(* Logix 5000 AddOnInstructionDefinition export Banner_Q5X_5000_Param_v4; software revision 33.00; part 2 of 3 *)
(* tags used below, declared in another part *)
   Q5X : Banner_Q5X_5000_v4;
   Port_Data : Banner_IOL_Port_v4;
   Port : DINT;
   Local_Control : DINT;
   Command_Being_Processed : BOOL;
   Update_Archive : BOOL;
   Index_Write_Inprocess : INT;
   Index_Write_Control : INT;
   Inprocess_Index : DINT;
(* Banner_Q5X_5000_Param_v4, continued *)

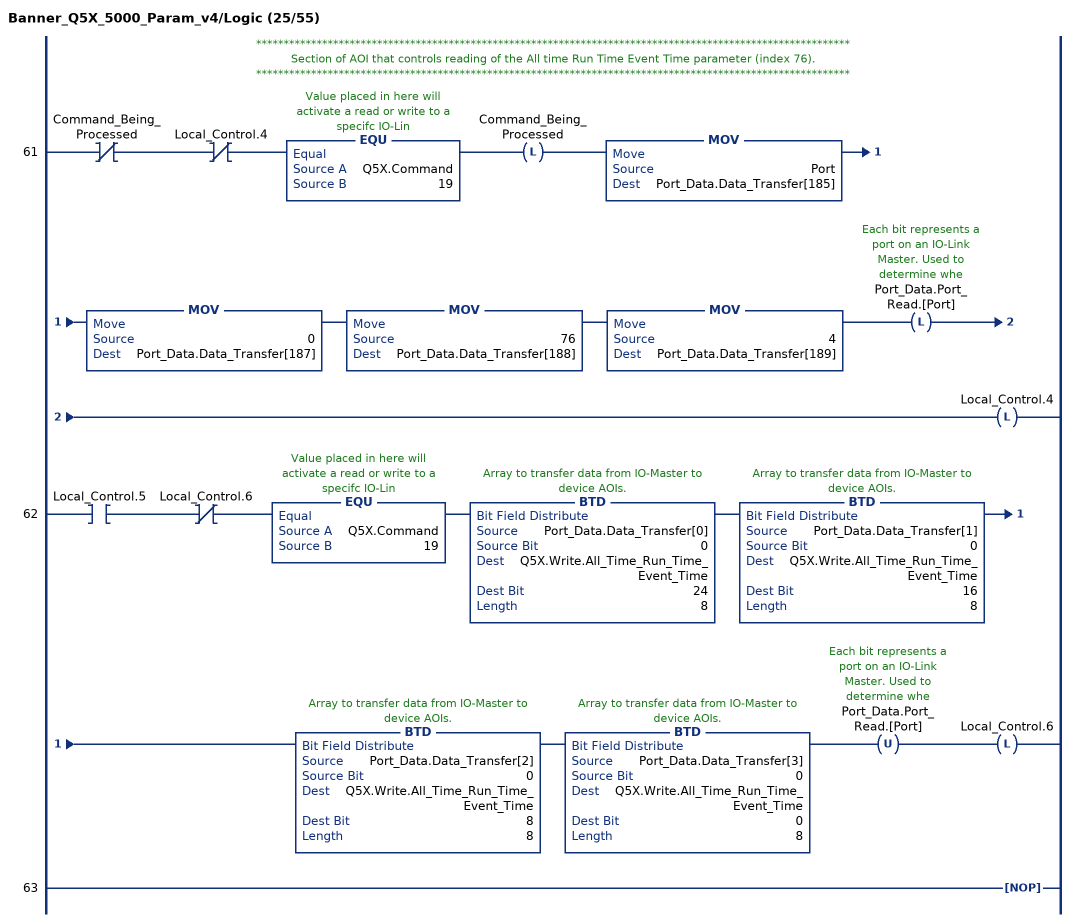
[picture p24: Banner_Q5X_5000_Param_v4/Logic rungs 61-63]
   // ************************************************************************************************************
   // Section of AOI that controls reading of the All time Run Time Event Time parameter (index 76).
   // ************************************************************************************************************
   61: XIO(Command_Being_Processed)XIO(Local_Control.4)EQU(Q5X.Command,19)OTL(Command_Being_Processed)MOV(Port,Port_Data.Data_Transfer[185])MOV(0,Port_Data.Data_Transfer[187])MOV(76,Port_Data.Data_Transfer[188])MOV(4,Port_Data.Data_Transfer[189])OTL(Port_Data.Port_Read.[Port])OTL(Local_Control.4);
   62: XIC(Local_Control.5)XIO(Local_Control.6)EQU(Q5X.Command,19)BTD(Port_Data.Data_Transfer[0],0,Q5X.Write.All_Time_Run_Time_Event_Time,24,8)BTD(Port_Data.Data_Transfer[1],0,Q5X.Write.All_Time_Run_Time_Event_Time,16,8)BTD(Port_Data.Data_Transfer[2],0,Q5X.Write.All_Time_Run_Time_Event_Time,8,8)BTD(Port_Data.Data_Transfer[3],0,Q5X.Write.All_Time_Run_Time_Event_Time,0,8)OTU(Port_Data.Port_Read.[Port])OTL(Local_Control.6);
   63: NOP();
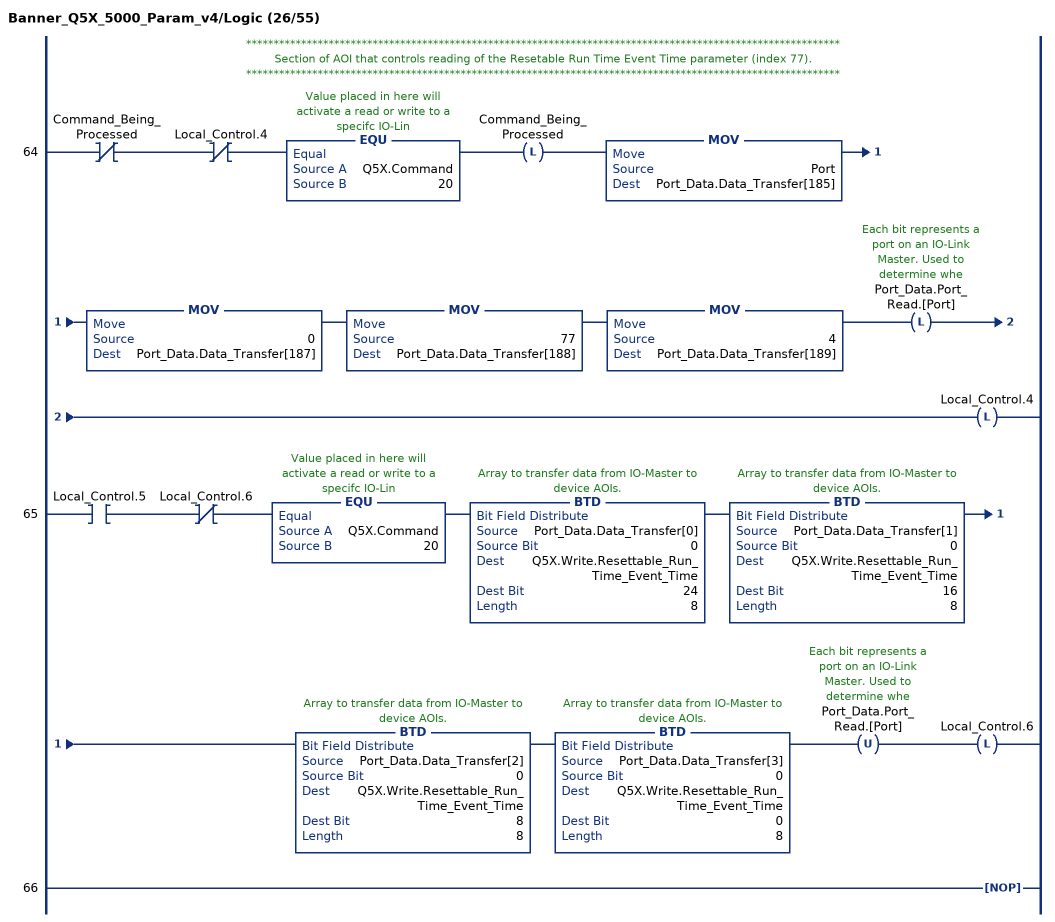
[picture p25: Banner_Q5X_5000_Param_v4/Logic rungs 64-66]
   // ************************************************************************************************************
   // Section of AOI that controls reading of the Resetable Run Time Event Time parameter (index 77).
   // ************************************************************************************************************
   64: XIO(Command_Being_Processed)XIO(Local_Control.4)EQU(Q5X.Command,20)OTL(Command_Being_Processed)MOV(Port,Port_Data.Data_Transfer[185])MOV(0,Port_Data.Data_Transfer[187])MOV(77,Port_Data.Data_Transfer[188])MOV(4,Port_Data.Data_Transfer[189])OTL(Port_Data.Port_Read.[Port])OTL(Local_Control.4);
   65: XIC(Local_Control.5)XIO(Local_Control.6)EQU(Q5X.Command,20)BTD(Port_Data.Data_Transfer[0],0,Q5X.Write.Resettable_Run_Time_Event_Time,24,8)BTD(Port_Data.Data_Transfer[1],0,Q5X.Write.Resettable_Run_Time_Event_Time,16,8)BTD(Port_Data.Data_Transfer[2],0,Q5X.Write.Resettable_Run_Time_Event_Time,8,8)BTD(Port_Data.Data_Transfer[3],0,Q5X.Write.Resettable_Run_Time_Event_Time,0,8)OTU(Port_Data.Port_Read.[Port])OTL(Local_Control.6);
   66: NOP();
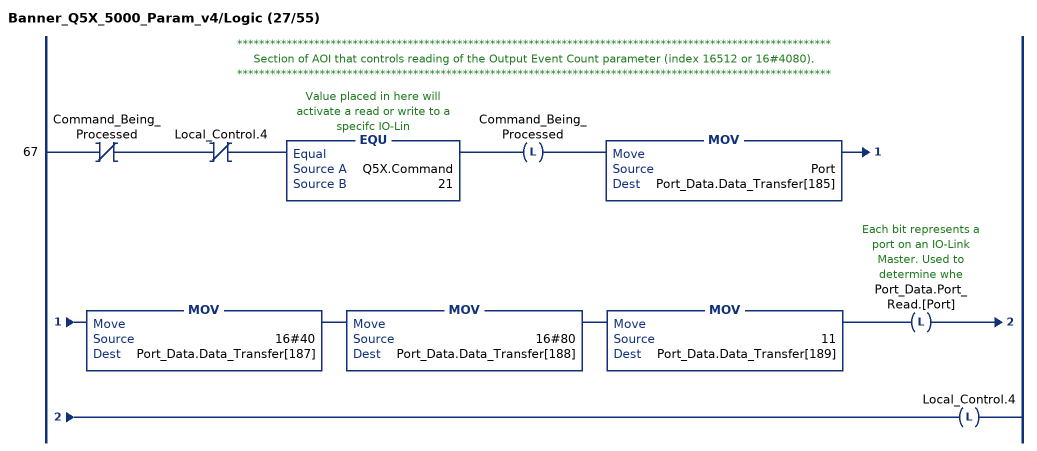
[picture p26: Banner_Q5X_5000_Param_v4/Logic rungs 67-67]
   // ************************************************************************************************************
   // Section of AOI that controls reading of the Output Event Count parameter (index 16512 or 16#4080).
   // ************************************************************************************************************
   67: XIO(Command_Being_Processed)XIO(Local_Control.4)EQU(Q5X.Command,21)OTL(Command_Being_Processed)MOV(Port,Port_Data.Data_Transfer[185])MOV(16#40,Port_Data.Data_Transfer[187])MOV(16#80,Port_Data.Data_Transfer[188])MOV(11,Port_Data.Data_Transfer[189])OTL(Port_Data.Port_Read.[Port])OTL(Local_Control.4);
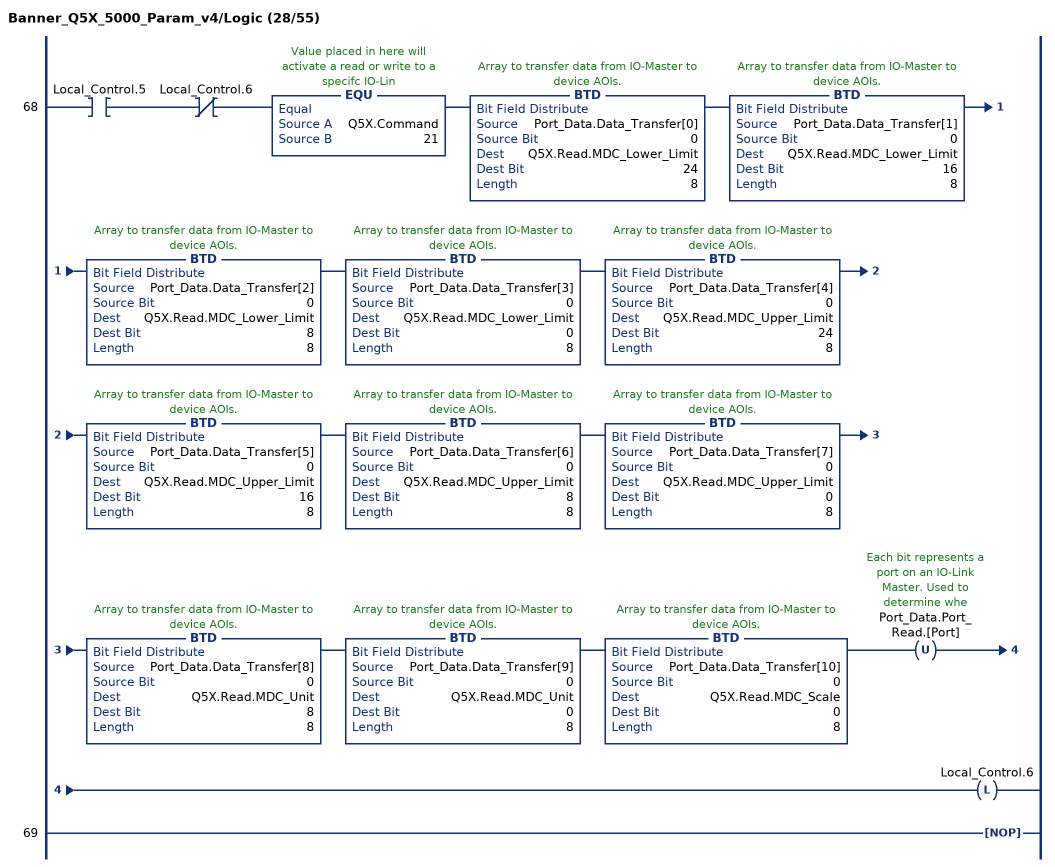
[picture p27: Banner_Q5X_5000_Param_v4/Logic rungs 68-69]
   68: XIC(Local_Control.5)XIO(Local_Control.6)EQU(Q5X.Command,21)BTD(Port_Data.Data_Transfer[0],0,Q5X.Read.MDC_Lower_Limit,24,8)BTD(Port_Data.Data_Transfer[1],0,Q5X.Read.MDC_Lower_Limit,16,8)BTD(Port_Data.Data_Transfer[2],0,Q5X.Read.MDC_Lower_Limit,8,8)BTD(Port_Data.Data_Transfer[3],0,Q5X.Read.MDC_Lower_Limit,0,8)BTD(Port_Data.Data_Transfer[4],0,Q5X.Read.MDC_Upper_Limit,24,8)BTD(Port_Data.Data_Transfer[5],0,Q5X.Read.MDC_Upper_Limit,16,8)BTD(Port_Data.Data_Transfer[6],0,Q5X.Read.MDC_Upper_Limit,8,8)BTD(Port_Data.Data_Transfer[7],0,Q5X.Read.MDC_Upper_Limit,0,8)BTD(Port_Data.Data_Transfer[8],0,Q5X.Read.MDC_Unit,8,8)BTD(Port_Data.Data_Transfer[9],0,Q5X.Read.MDC_Unit,0,8)BTD(Port_Data.Data_Transfer[10],0,Q5X.Read.MDC_Scale,0,8)OTU(Port_Data.Port_Read.[Port])OTL(Local_Control.6);
   69: NOP();
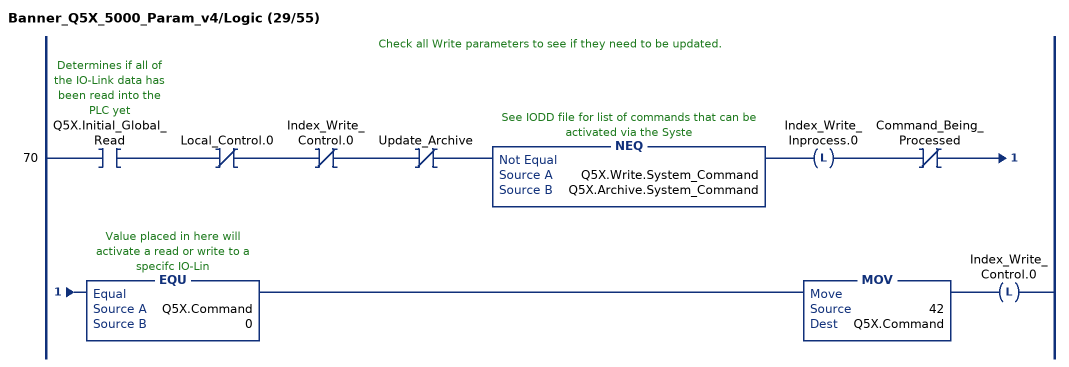
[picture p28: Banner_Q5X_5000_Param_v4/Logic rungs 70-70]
   // Check all Write parameters to see if they need to be updated.
   70: XIC(Q5X.Initial_Global_Read)XIO(Local_Control.0)XIO(Index_Write_Control.0)XIO(Update_Archive)NEQ(Q5X.Write.System_Command,Q5X.Archive.System_Command)OTL(Index_Write_Inprocess.0)XIO(Command_Being_Processed)EQU(Q5X.Command,0)MOV(42,Q5X.Command)OTL(Index_Write_Control.0);
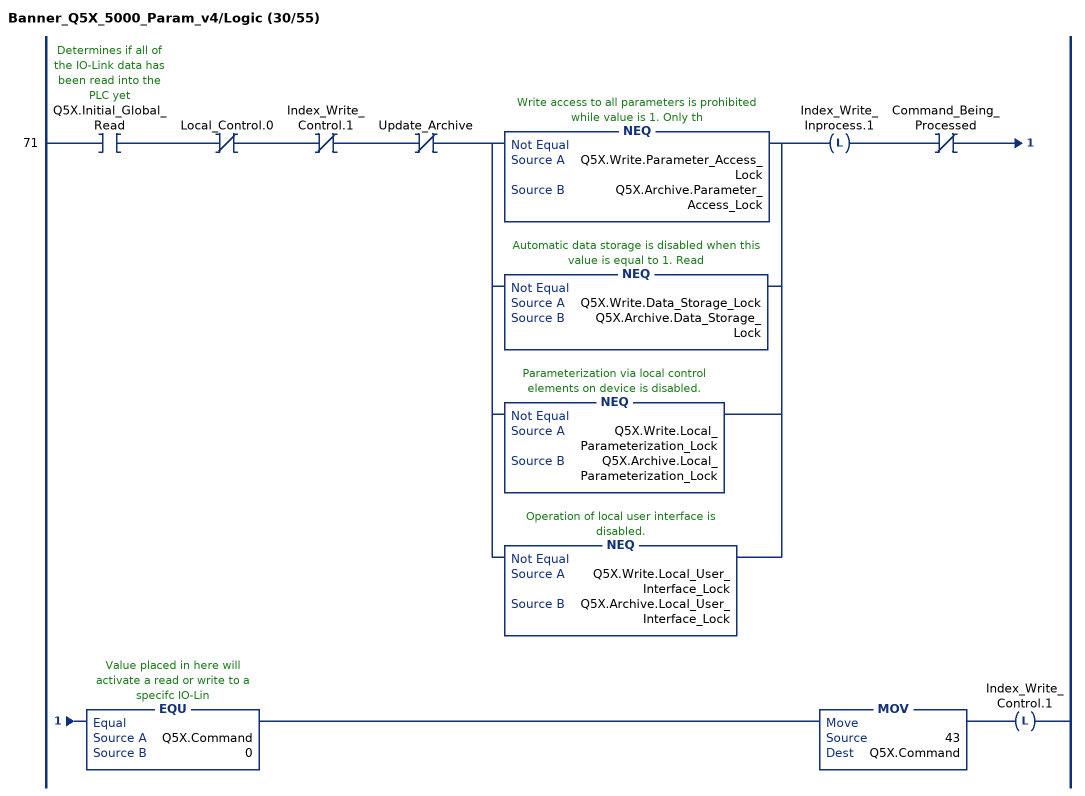
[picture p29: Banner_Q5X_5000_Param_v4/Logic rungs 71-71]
   71: XIC(Q5X.Initial_Global_Read)XIO(Local_Control.0)XIO(Index_Write_Control.1)XIO(Update_Archive)[NEQ(Q5X.Write.Parameter_Access_Lock,Q5X.Archive.Parameter_Access_Lock) ,NEQ(Q5X.Write.Data_Storage_Lock,Q5X.Archive.Data_Storage_Lock) ,NEQ(Q5X.Write.Local_Parameterization_Lock,Q5X.Archive.Local_Parameterization_Lock) ,NEQ(Q5X.Write.Local_User_Interface_Lock,Q5X.Archive.Local_User_Interface_Lock) ]OTL(Index_Write_Inprocess.1)XIO(Command_Being_Processed)EQU(Q5X.Command,0)MOV(43,Q5X.Command)OTL(Index_Write_Control.1);
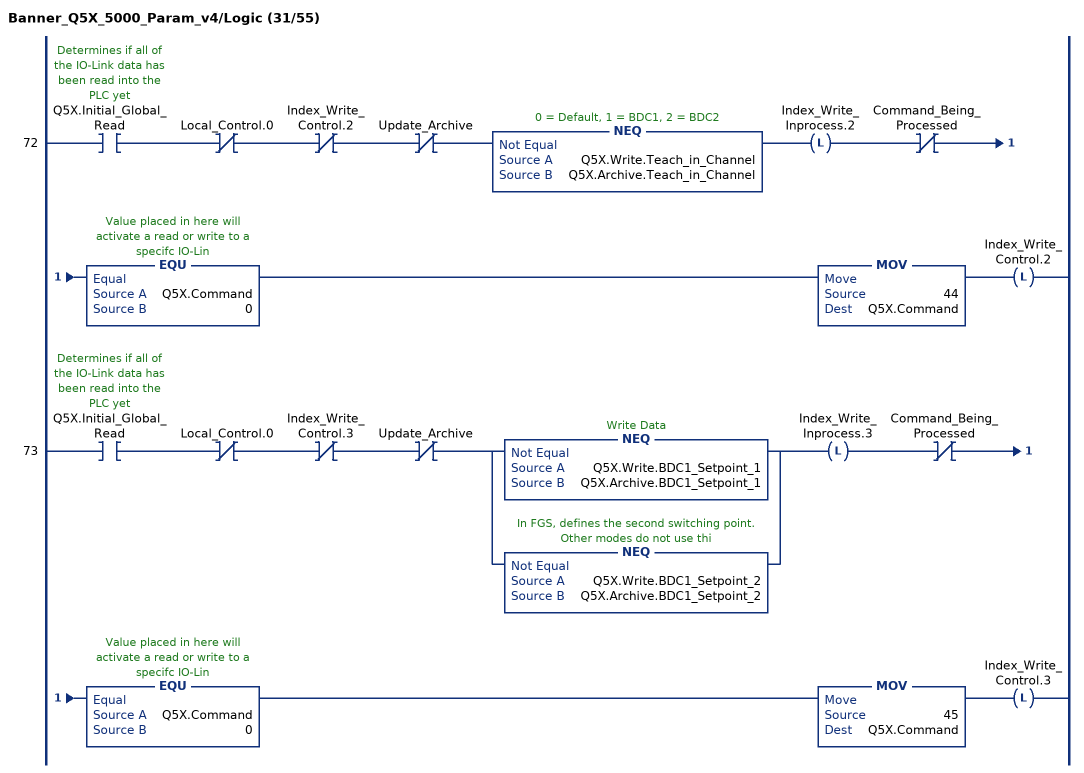
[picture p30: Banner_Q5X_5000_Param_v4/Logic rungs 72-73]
   72: XIC(Q5X.Initial_Global_Read)XIO(Local_Control.0)XIO(Index_Write_Control.2)XIO(Update_Archive)NEQ(Q5X.Write.Teach_in_Channel,Q5X.Archive.Teach_in_Channel)OTL(Index_Write_Inprocess.2)XIO(Command_Being_Processed)EQU(Q5X.Command,0)MOV(44,Q5X.Command)OTL(Index_Write_Control.2);
   73: XIC(Q5X.Initial_Global_Read)XIO(Local_Control.0)XIO(Index_Write_Control.3)XIO(Update_Archive)[NEQ(Q5X.Write.BDC1_Setpoint_1,Q5X.Archive.BDC1_Setpoint_1) ,NEQ(Q5X.Write.BDC1_Setpoint_2,Q5X.Archive.BDC1_Setpoint_2) ]OTL(Index_Write_Inprocess.3)XIO(Command_Being_Processed)EQU(Q5X.Command,0)MOV(45,Q5X.Command)OTL(Index_Write_Control.3);
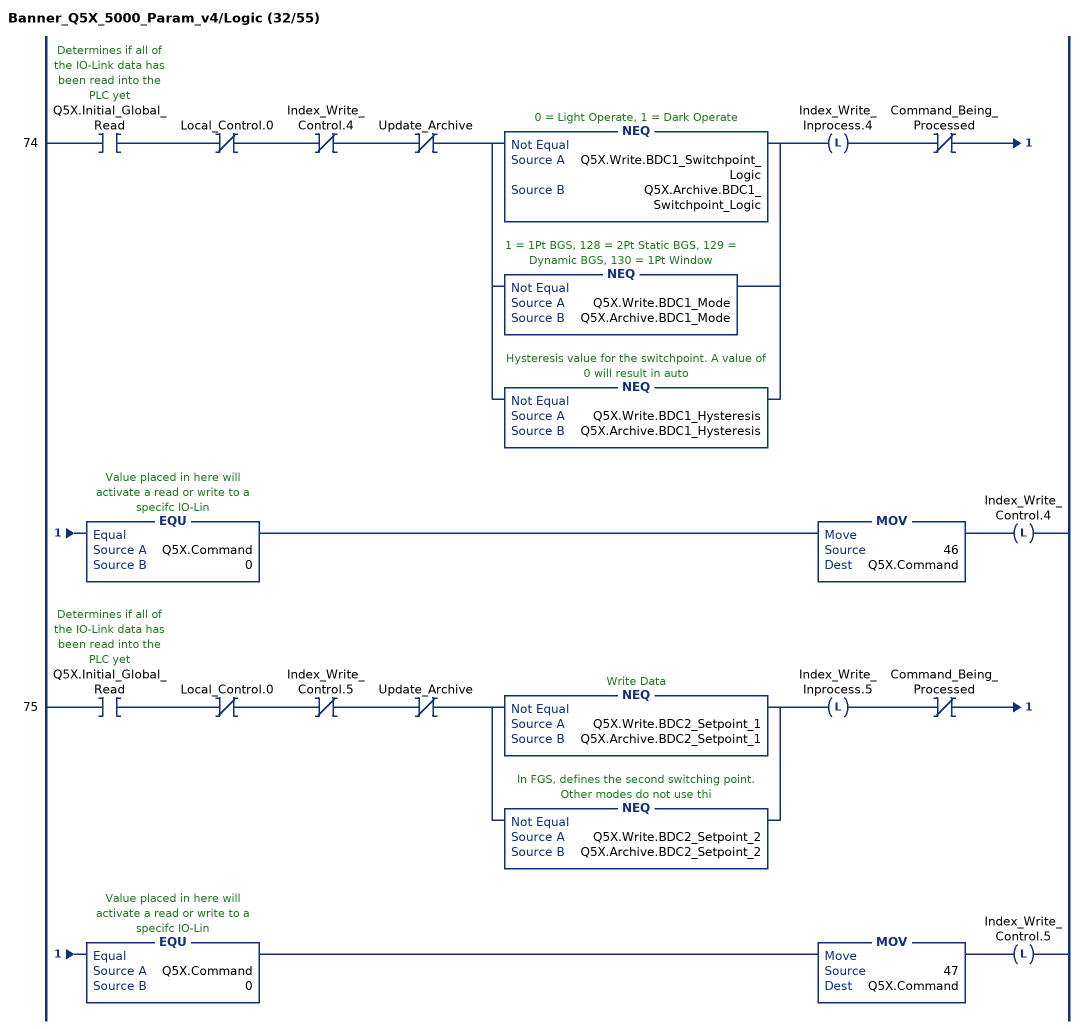
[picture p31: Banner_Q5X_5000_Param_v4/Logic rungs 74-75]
   74: XIC(Q5X.Initial_Global_Read)XIO(Local_Control.0)XIO(Index_Write_Control.4)XIO(Update_Archive)[NEQ(Q5X.Write.BDC1_Switchpoint_Logic,Q5X.Archive.BDC1_Switchpoint_Logic) ,NEQ(Q5X.Write.BDC1_Mode,Q5X.Archive.BDC1_Mode) ,NEQ(Q5X.Write.BDC1_Hysteresis,Q5X.Archive.BDC1_Hysteresis) ]OTL(Index_Write_Inprocess.4)XIO(Command_Being_Processed)EQU(Q5X.Command,0)MOV(46,Q5X.Command)OTL(Index_Write_Control.4);
   75: XIC(Q5X.Initial_Global_Read)XIO(Local_Control.0)XIO(Index_Write_Control.5)XIO(Update_Archive)[NEQ(Q5X.Write.BDC2_Setpoint_1,Q5X.Archive.BDC2_Setpoint_1) ,NEQ(Q5X.Write.BDC2_Setpoint_2,Q5X.Archive.BDC2_Setpoint_2) ]OTL(Index_Write_Inprocess.5)XIO(Command_Being_Processed)EQU(Q5X.Command,0)MOV(47,Q5X.Command)OTL(Index_Write_Control.5);
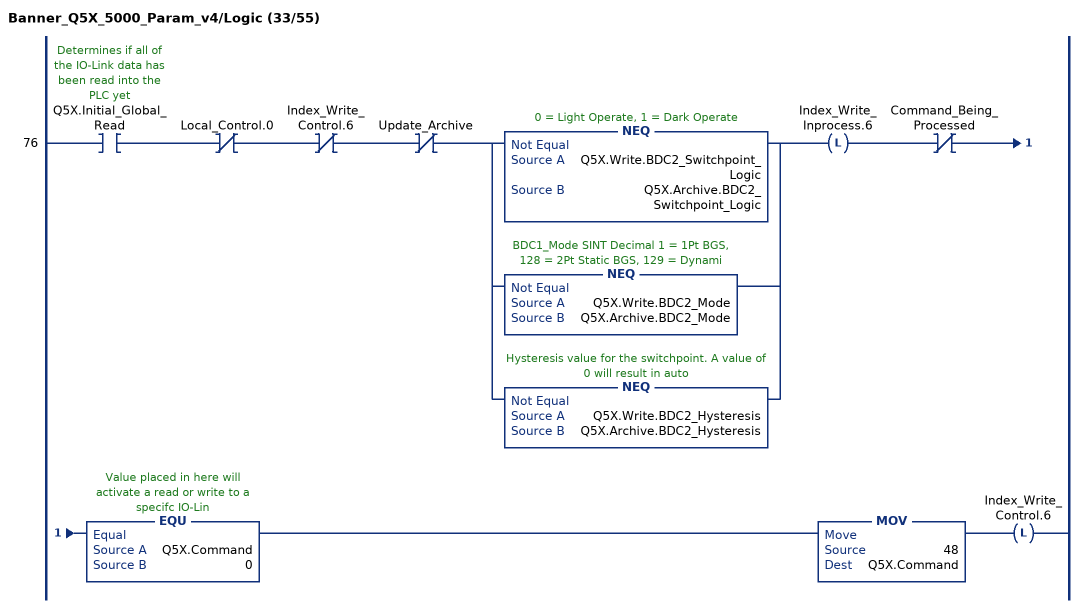
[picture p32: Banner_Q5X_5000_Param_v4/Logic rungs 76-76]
   76: XIC(Q5X.Initial_Global_Read)XIO(Local_Control.0)XIO(Index_Write_Control.6)XIO(Update_Archive)[NEQ(Q5X.Write.BDC2_Switchpoint_Logic,Q5X.Archive.BDC2_Switchpoint_Logic) ,NEQ(Q5X.Write.BDC2_Mode,Q5X.Archive.BDC2_Mode) ,NEQ(Q5X.Write.BDC2_Hysteresis,Q5X.Archive.BDC2_Hysteresis) ]OTL(Index_Write_Inprocess.6)XIO(Command_Being_Processed)EQU(Q5X.Command,0)MOV(48,Q5X.Command)OTL(Index_Write_Control.6);
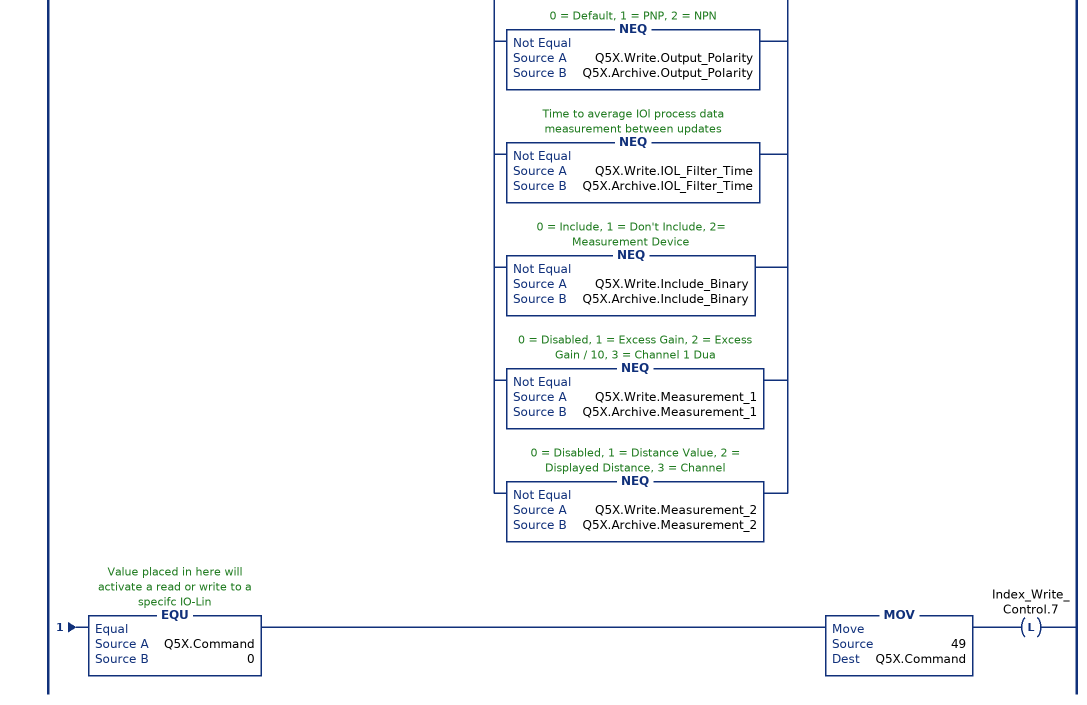
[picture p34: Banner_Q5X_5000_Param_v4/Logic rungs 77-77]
   77: XIC(Q5X.Initial_Global_Read)XIO(Local_Control.0)XIO(Index_Write_Control.7)XIO(Update_Archive)[NEQ(Q5X.Write.Response_Speed,Q5X.Archive.Response_Speed) ,NEQ(Q5X.Write.Gain,Q5X.Archive.Gain) ,NEQ(Q5X.Write.Secondary_Output_Mode,Q5X.Archive.Secondary_Output_Mode) ,NEQ(Q5X.Write.Zero_Reference_Location,Q5X.Archive.Zero_Reference_Location) ,NEQ(Q5X.Write.Shift_Zero_after_Teach,Q5X.Archive.Shift_Zero_after_Teach) ,NEQ(Q5X.Write.Display_Read,Q5X.Archive.Display_Read) ,NEQ(Q5X.Write.Display_Units,Q5X.Archive.Display_Units) ,NEQ(Q5X.Write.Pushbutton_Lockout,Q5X.Archive.Pushbutton_Lockout) ,NEQ(Q5X.Write.Output_Polarity,Q5X.Archive.Output_Polarity) ,NEQ(Q5X.Write.IOL_Filter_Time,Q5X.Archive.IOL_Filter_Time) ,NEQ(Q5X.Write.Include_Binary,Q5X.Archive.Include_Binary) ,NEQ(Q5X.Write.Measurement_1,Q5X.Archive.Measurement_1) ,NEQ(Q5X.Write.Measurement_2,Q5X.Archive.Measurement_2) ]OTL(Index_Write_Inprocess.7)XIO(Command_Being_Processed)EQU(Q5X.Command,0)MOV(49,Q5X.Command)OTL(Index_Write_Control.7);
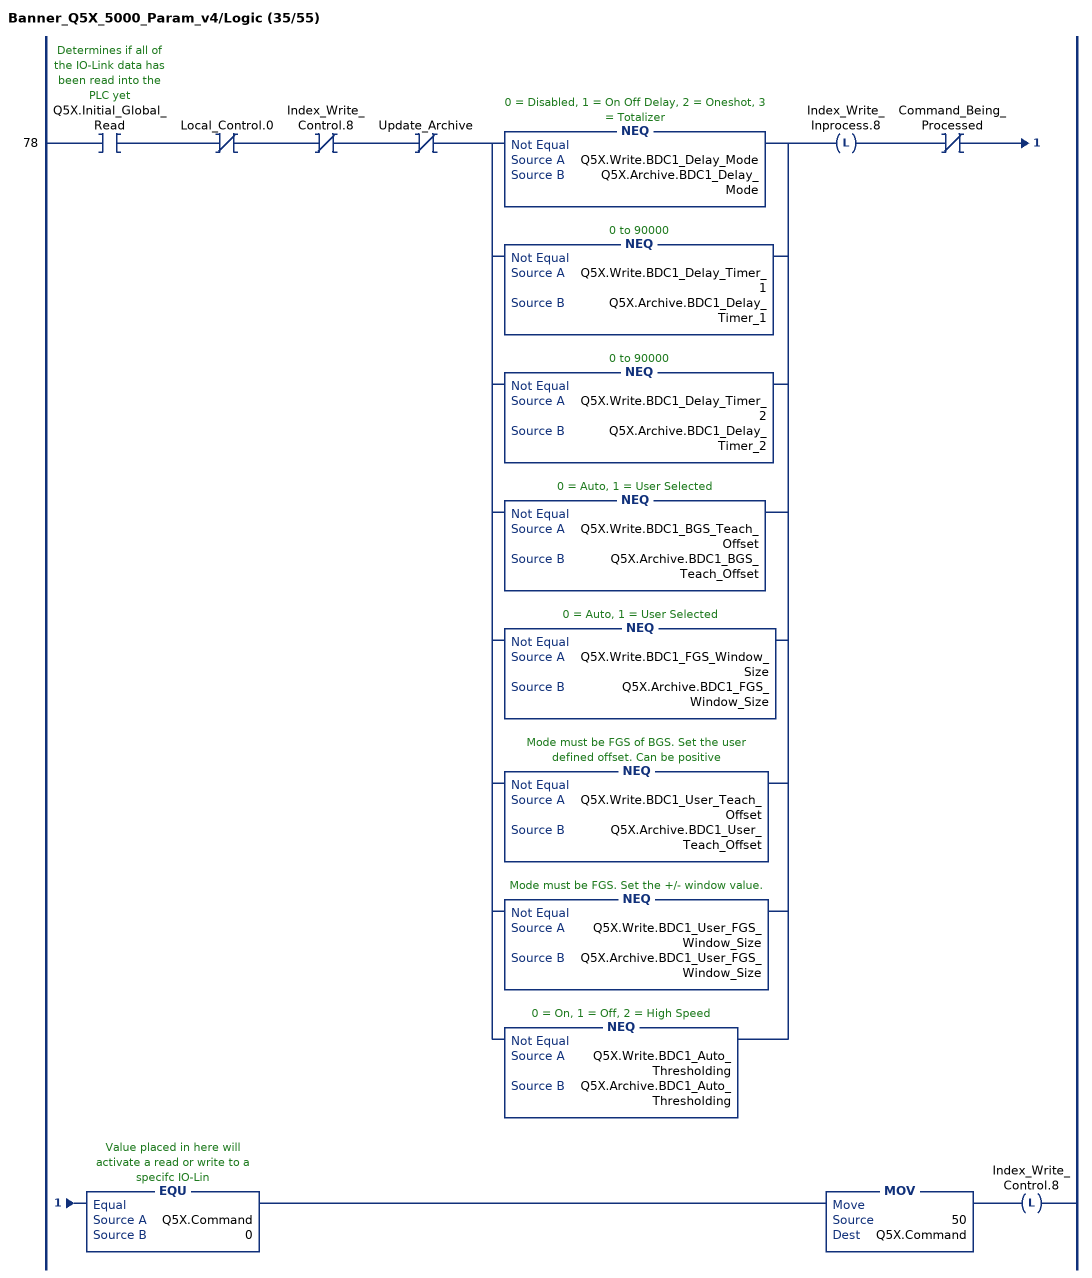
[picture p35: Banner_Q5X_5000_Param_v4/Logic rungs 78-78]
   78: XIC(Q5X.Initial_Global_Read)XIO(Local_Control.0)XIO(Index_Write_Control.8)XIO(Update_Archive)[NEQ(Q5X.Write.BDC1_Delay_Mode,Q5X.Archive.BDC1_Delay_Mode) ,NEQ(Q5X.Write.BDC1_Delay_Timer_1,Q5X.Archive.BDC1_Delay_Timer_1) ,NEQ(Q5X.Write.BDC1_Delay_Timer_2,Q5X.Archive.BDC1_Delay_Timer_2) ,NEQ(Q5X.Write.BDC1_BGS_Teach_Offset,Q5X.Archive.BDC1_BGS_Teach_Offset) ,NEQ(Q5X.Write.BDC1_FGS_Window_Size,Q5X.Archive.BDC1_FGS_Window_Size) ,NEQ(Q5X.Write.BDC1_User_Teach_Offset,Q5X.Archive.BDC1_User_Teach_Offset) ,NEQ(Q5X.Write.BDC1_User_FGS_Window_Size,Q5X.Archive.BDC1_User_FGS_Window_Size) ,NEQ(Q5X.Write.BDC1_Auto_Thresholding,Q5X.Archive.BDC1_Auto_Thresholding) ]OTL(Index_Write_Inprocess.8)XIO(Command_Being_Processed)EQU(Q5X.Command,0)MOV(50,Q5X.Command)OTL(Index_Write_Control.8);
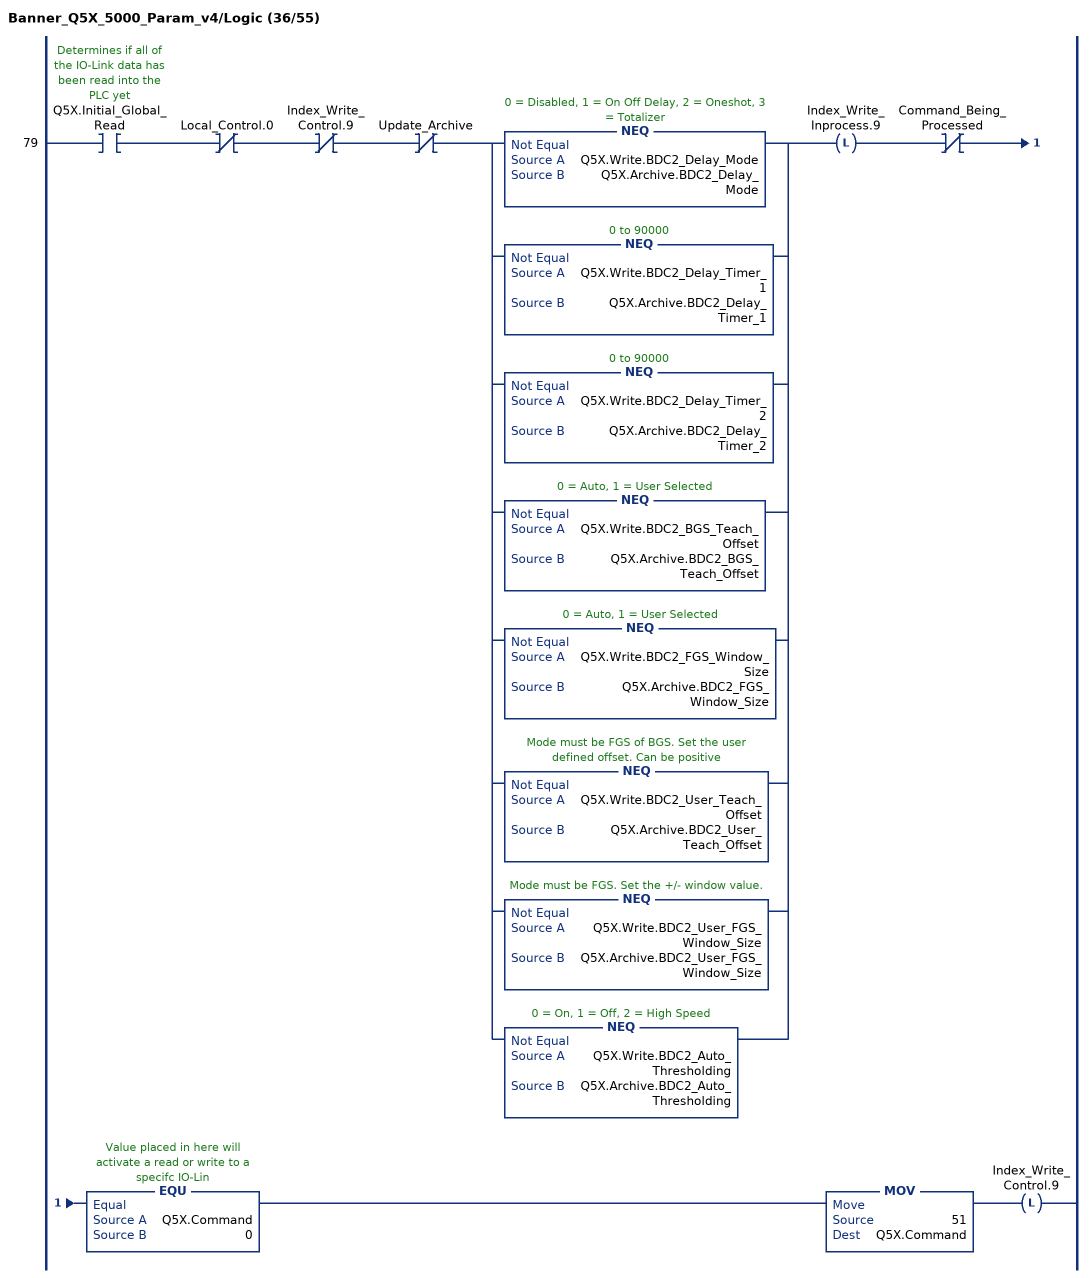
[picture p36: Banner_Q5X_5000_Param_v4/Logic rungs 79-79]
   79: XIC(Q5X.Initial_Global_Read)XIO(Local_Control.0)XIO(Index_Write_Control.9)XIO(Update_Archive)[NEQ(Q5X.Write.BDC2_Delay_Mode,Q5X.Archive.BDC2_Delay_Mode) ,NEQ(Q5X.Write.BDC2_Delay_Timer_1,Q5X.Archive.BDC2_Delay_Timer_1) ,NEQ(Q5X.Write.BDC2_Delay_Timer_2,Q5X.Archive.BDC2_Delay_Timer_2) ,NEQ(Q5X.Write.BDC2_BGS_Teach_Offset,Q5X.Archive.BDC2_BGS_Teach_Offset) ,NEQ(Q5X.Write.BDC2_FGS_Window_Size,Q5X.Archive.BDC2_FGS_Window_Size) ,NEQ(Q5X.Write.BDC2_User_Teach_Offset,Q5X.Archive.BDC2_User_Teach_Offset) ,NEQ(Q5X.Write.BDC2_User_FGS_Window_Size,Q5X.Archive.BDC2_User_FGS_Window_Size) ,NEQ(Q5X.Write.BDC2_Auto_Thresholding,Q5X.Archive.BDC2_Auto_Thresholding) ]OTL(Index_Write_Inprocess.9)XIO(Command_Being_Processed)EQU(Q5X.Command,0)MOV(51,Q5X.Command)OTL(Index_Write_Control.9);
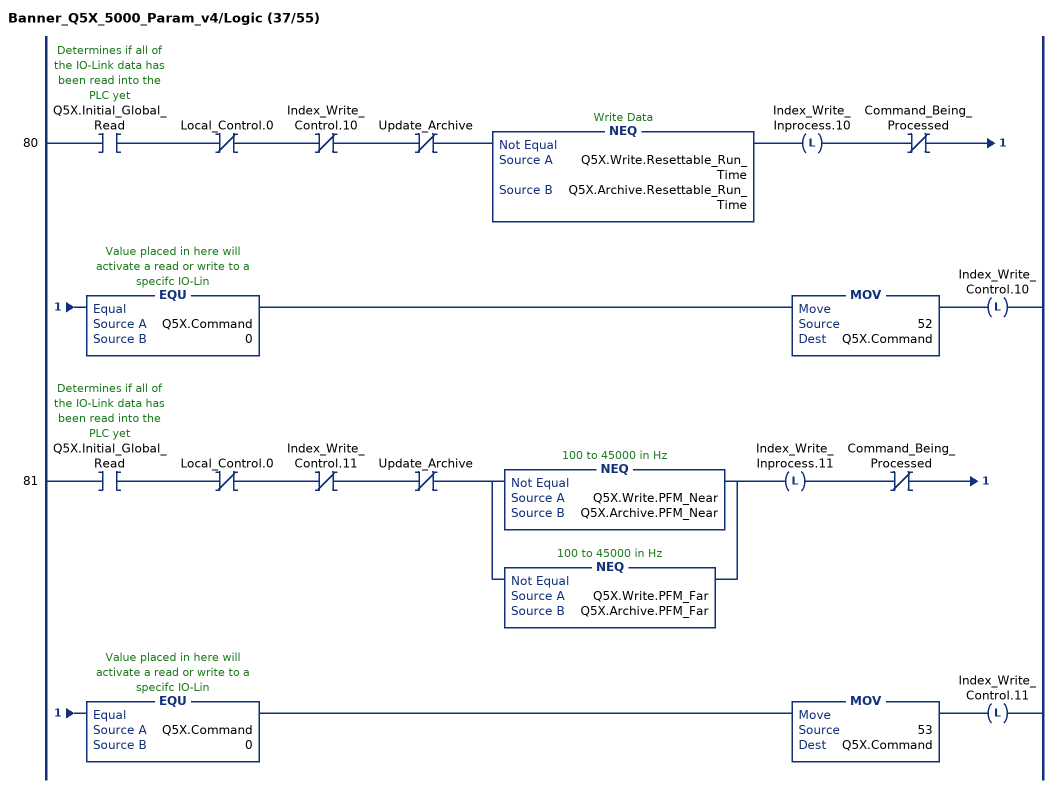
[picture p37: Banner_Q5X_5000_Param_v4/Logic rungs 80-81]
   80: XIC(Q5X.Initial_Global_Read)XIO(Local_Control.0)XIO(Index_Write_Control.10)XIO(Update_Archive)NEQ(Q5X.Write.Resettable_Run_Time,Q5X.Archive.Resettable_Run_Time)OTL(Index_Write_Inprocess.10)XIO(Command_Being_Processed)EQU(Q5X.Command,0)MOV(52,Q5X.Command)OTL(Index_Write_Control.10);
   81: XIC(Q5X.Initial_Global_Read)XIO(Local_Control.0)XIO(Index_Write_Control.11)XIO(Update_Archive)[NEQ(Q5X.Write.PFM_Near,Q5X.Archive.PFM_Near) ,NEQ(Q5X.Write.PFM_Far,Q5X.Archive.PFM_Far) ]OTL(Index_Write_Inprocess.11)XIO(Command_Being_Processed)EQU(Q5X.Command,0)MOV(53,Q5X.Command)OTL(Index_Write_Control.11);
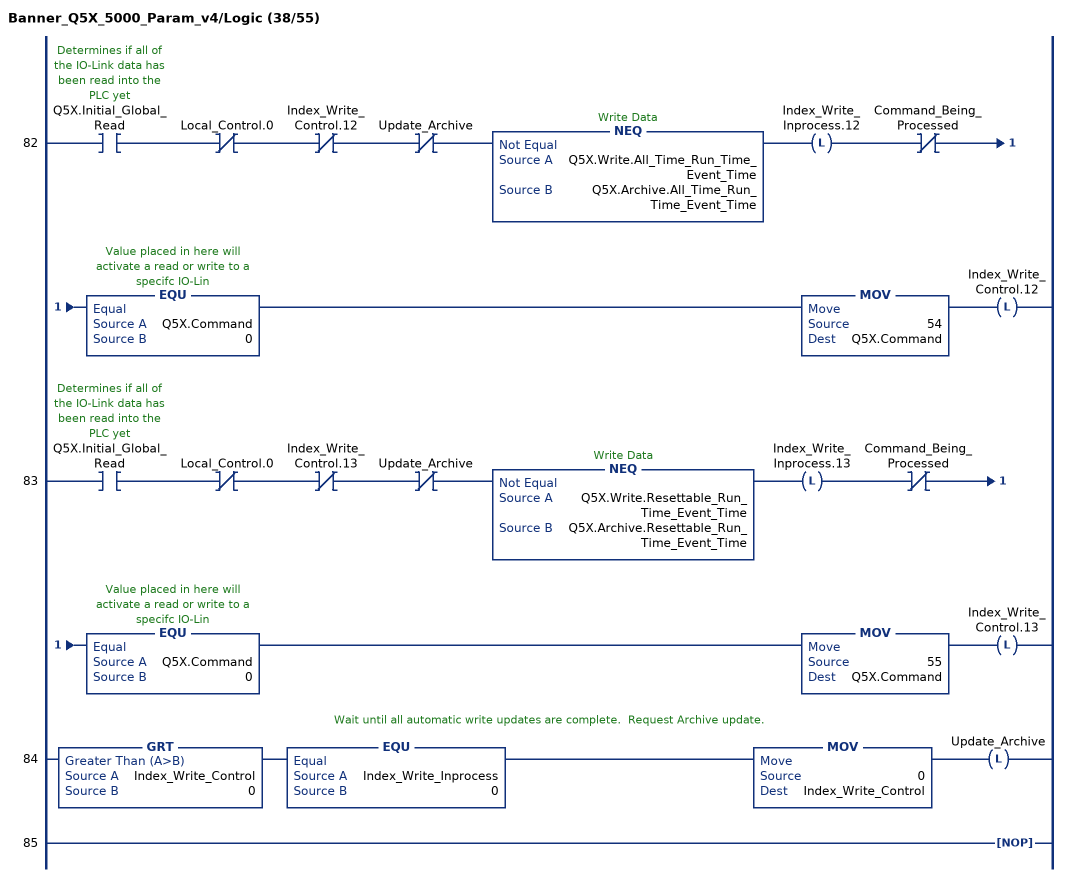
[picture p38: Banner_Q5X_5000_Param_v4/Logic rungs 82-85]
   82: XIC(Q5X.Initial_Global_Read)XIO(Local_Control.0)XIO(Index_Write_Control.12)XIO(Update_Archive)NEQ(Q5X.Write.All_Time_Run_Time_Event_Time,Q5X.Archive.All_Time_Run_Time_Event_Time)OTL(Index_Write_Inprocess.12)XIO(Command_Being_Processed)EQU(Q5X.Command,0)MOV(54,Q5X.Command)OTL(Index_Write_Control.12);
   83: XIC(Q5X.Initial_Global_Read)XIO(Local_Control.0)XIO(Index_Write_Control.13)XIO(Update_Archive)NEQ(Q5X.Write.Resettable_Run_Time_Event_Time,Q5X.Archive.Resettable_Run_Time_Event_Time)OTL(Index_Write_Inprocess.13)XIO(Command_Being_Processed)EQU(Q5X.Command,0)MOV(55,Q5X.Command)OTL(Index_Write_Control.13);
   // Wait until all automatic write updates are complete.  Request Archive update.
   84: GRT(Index_Write_Control,0)EQU(Index_Write_Inprocess,0)MOV(0,Index_Write_Control)OTL(Update_Archive);
   85: NOP();
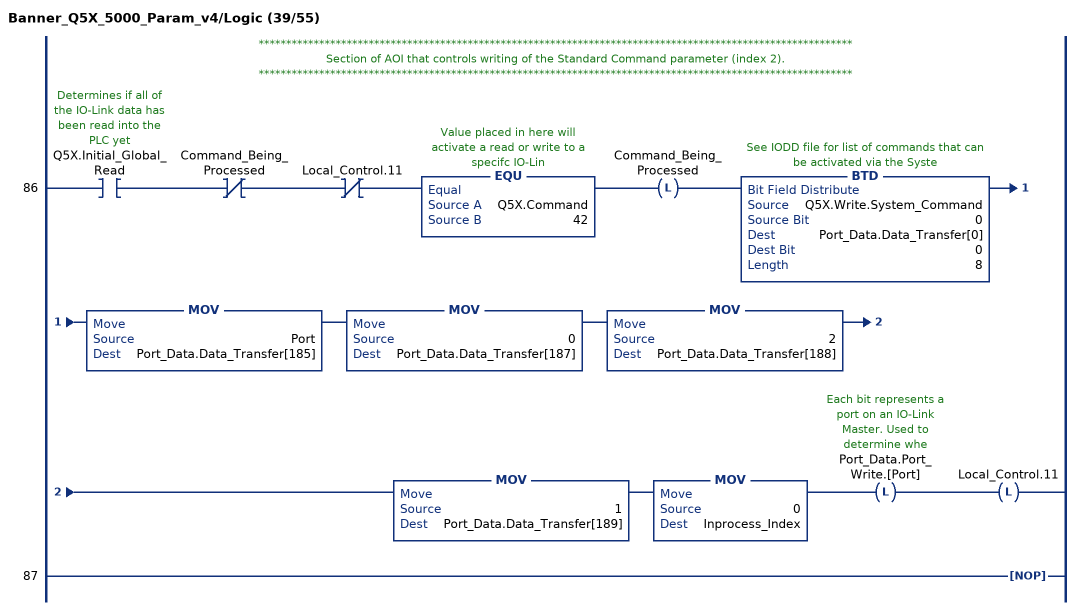
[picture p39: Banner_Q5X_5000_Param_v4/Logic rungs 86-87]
   // ************************************************************************************************************
   // Section of AOI that controls writing of the Standard Command parameter (index 2).
   // ************************************************************************************************************
   86: XIC(Q5X.Initial_Global_Read)XIO(Command_Being_Processed)XIO(Local_Control.11)EQU(Q5X.Command,42)OTL(Command_Being_Processed)BTD(Q5X.Write.System_Command,0,Port_Data.Data_Transfer[0],0,8)MOV(Port,Port_Data.Data_Transfer[185])MOV(0,Port_Data.Data_Transfer[187])MOV(2,Port_Data.Data_Transfer[188])MOV(1,Port_Data.Data_Transfer[189])MOV(0,Inprocess_Index)OTL(Port_Data.Port_Write.[Port])OTL(Local_Control.11);
   87: NOP();
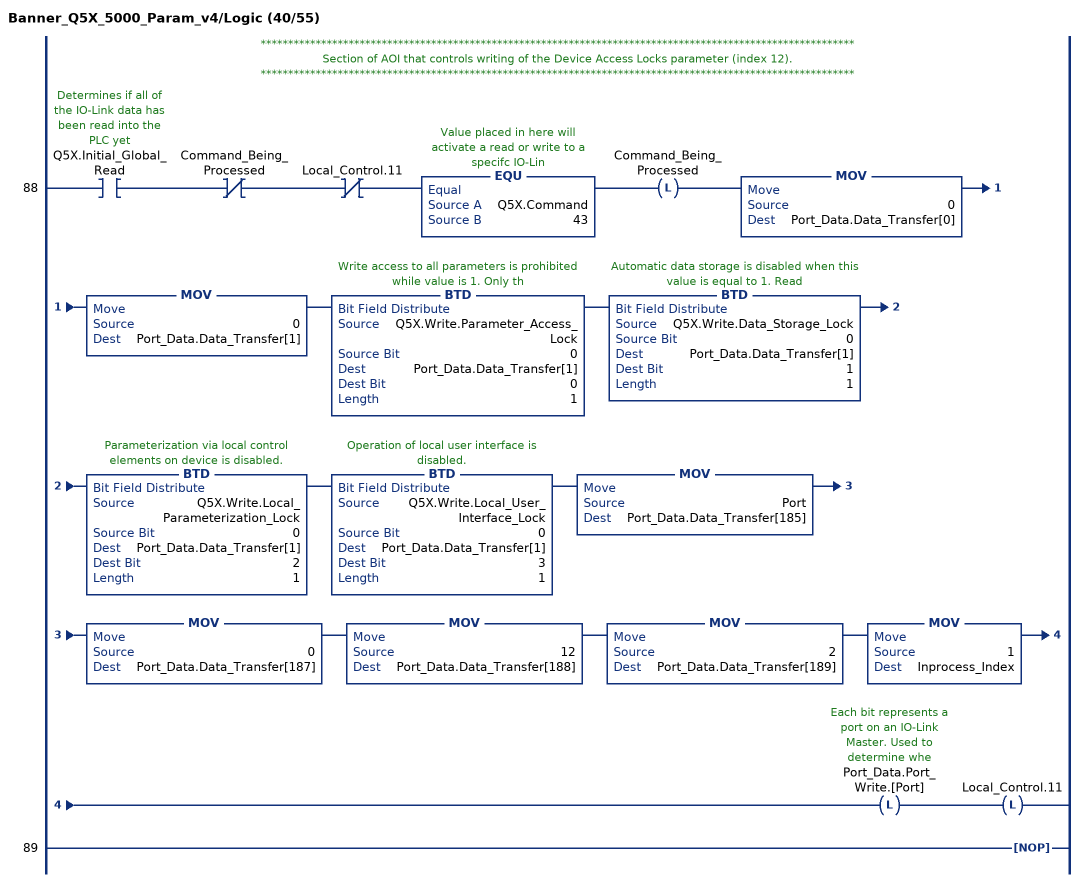
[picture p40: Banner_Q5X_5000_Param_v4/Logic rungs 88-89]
   // ************************************************************************************************************
   // Section of AOI that controls writing of the Device Access Locks parameter (index 12).
   // ************************************************************************************************************
   88: XIC(Q5X.Initial_Global_Read)XIO(Command_Being_Processed)XIO(Local_Control.11)EQU(Q5X.Command,43)OTL(Command_Being_Processed)MOV(0,Port_Data.Data_Transfer[0])MOV(0,Port_Data.Data_Transfer[1])BTD(Q5X.Write.Parameter_Access_Lock,0,Port_Data.Data_Transfer[1],0,1)BTD(Q5X.Write.Data_Storage_Lock,0,Port_Data.Data_Transfer[1],1,1)BTD(Q5X.Write.Local_Parameterization_Lock,0,Port_Data.Data_Transfer[1],2,1)BTD(Q5X.Write.Local_User_Interface_Lock,0,Port_Data.Data_Transfer[1],3,1)MOV(Port,Port_Data.Data_Transfer[185])MOV(0,Port_Data.Data_Transfer[187])MOV(12,Port_Data.Data_Transfer[188])MOV(2,Port_Data.Data_Transfer[189])MOV(1,Inprocess_Index)OTL(Port_Data.Port_Write.[Port])OTL(Local_Control.11);
   89: NOP();
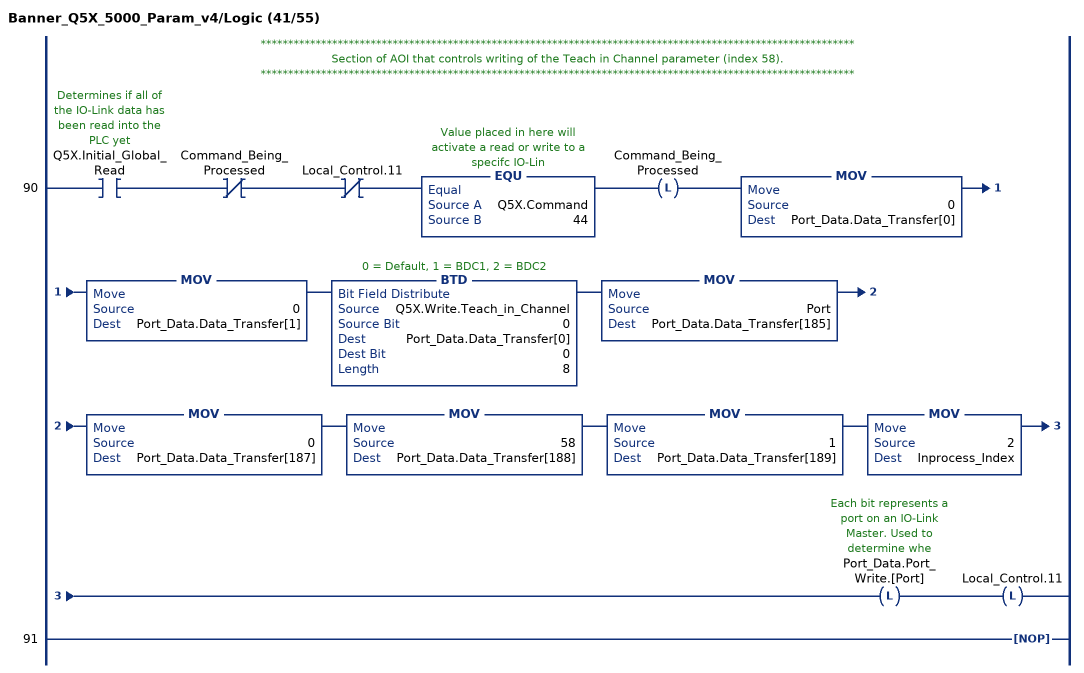
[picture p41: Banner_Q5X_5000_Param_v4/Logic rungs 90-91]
   // ************************************************************************************************************
   // Section of AOI that controls writing of the Teach in Channel parameter (index 58).
   // ************************************************************************************************************
   90: XIC(Q5X.Initial_Global_Read)XIO(Command_Being_Processed)XIO(Local_Control.11)EQU(Q5X.Command,44)OTL(Command_Being_Processed)MOV(0,Port_Data.Data_Transfer[0])MOV(0,Port_Data.Data_Transfer[1])BTD(Q5X.Write.Teach_in_Channel,0,Port_Data.Data_Transfer[0],0,8)MOV(Port,Port_Data.Data_Transfer[185])MOV(0,Port_Data.Data_Transfer[187])MOV(58,Port_Data.Data_Transfer[188])MOV(1,Port_Data.Data_Transfer[189])MOV(2,Inprocess_Index)OTL(Port_Data.Port_Write.[Port])OTL(Local_Control.11);
   91: NOP();
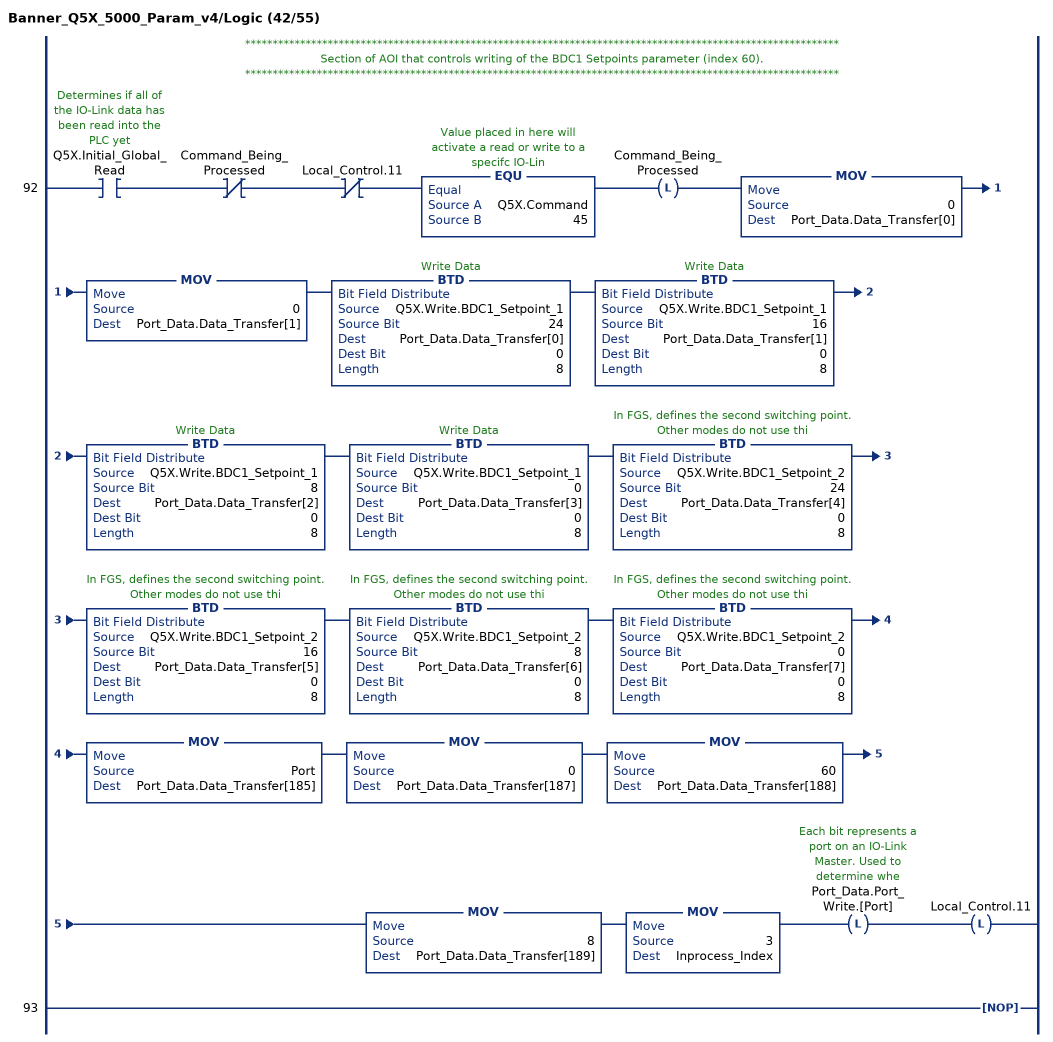
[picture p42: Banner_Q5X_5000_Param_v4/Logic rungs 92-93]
   // ************************************************************************************************************
   // Section of AOI that controls writing of the BDC1 Setpoints parameter (index 60).
   // ************************************************************************************************************
   92: XIC(Q5X.Initial_Global_Read)XIO(Command_Being_Processed)XIO(Local_Control.11)EQU(Q5X.Command,45)OTL(Command_Being_Processed)MOV(0,Port_Data.Data_Transfer[0])MOV(0,Port_Data.Data_Transfer[1])BTD(Q5X.Write.BDC1_Setpoint_1,24,Port_Data.Data_Transfer[0],0,8)BTD(Q5X.Write.BDC1_Setpoint_1,16,Port_Data.Data_Transfer[1],0,8)BTD(Q5X.Write.BDC1_Setpoint_1,8,Port_Data.Data_Transfer[2],0,8)BTD(Q5X.Write.BDC1_Setpoint_1,0,Port_Data.Data_Transfer[3],0,8)BTD(Q5X.Write.BDC1_Setpoint_2,24,Port_Data.Data_Transfer[4],0,8)BTD(Q5X.Write.BDC1_Setpoint_2,16,Port_Data.Data_Transfer[5],0,8)BTD(Q5X.Write.BDC1_Setpoint_2,8,Port_Data.Data_Transfer[6],0,8)BTD(Q5X.Write.BDC1_Setpoint_2,0,Port_Data.Data_Transfer[7],0,8)MOV(Port,Port_Data.Data_Transfer[185])MOV(0,Port_Data.Data_Transfer[187])MOV(60,Port_Data.Data_Transfer[188])MOV(8,Port_Data.Data_Transfer[189])MOV(3,Inprocess_Index)OTL(Port_Data.Port_Write.[Port])OTL(Local_Control.11);
   93: NOP();
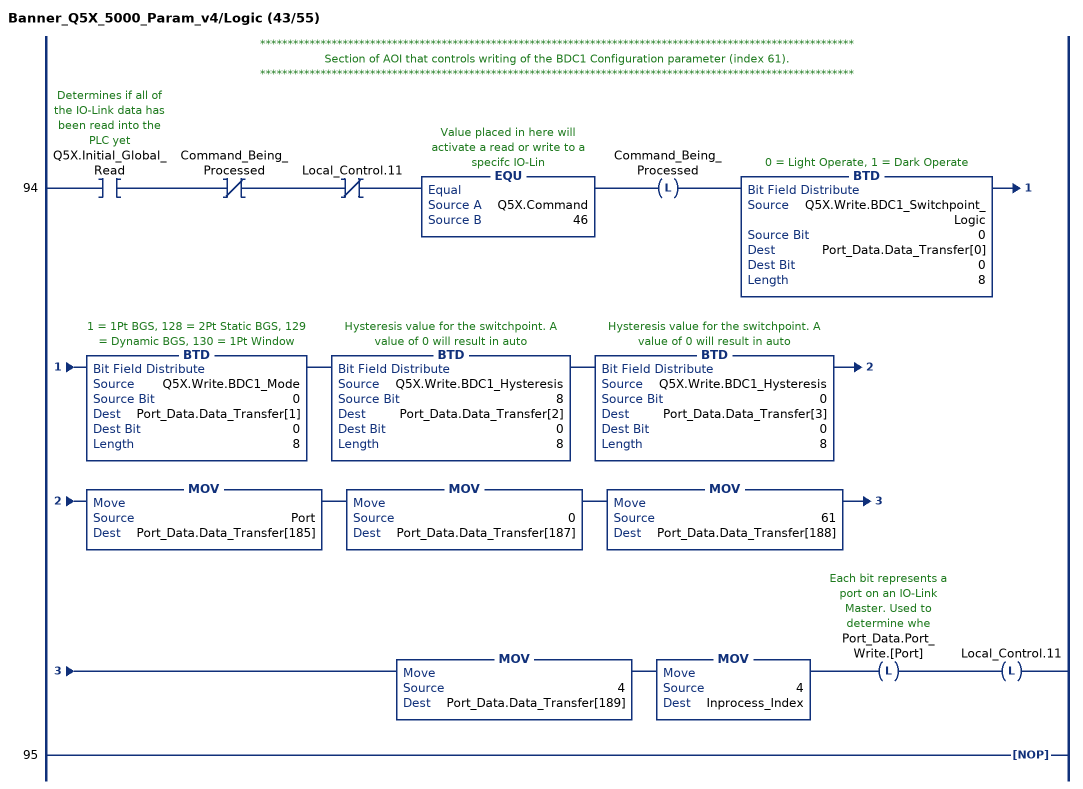
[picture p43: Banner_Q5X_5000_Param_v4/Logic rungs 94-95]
   // ************************************************************************************************************
   // Section of AOI that controls writing of the BDC1 Configuration parameter (index 61).
   // ************************************************************************************************************
   94: XIC(Q5X.Initial_Global_Read)XIO(Command_Being_Processed)XIO(Local_Control.11)EQU(Q5X.Command,46)OTL(Command_Being_Processed)BTD(Q5X.Write.BDC1_Switchpoint_Logic,0,Port_Data.Data_Transfer[0],0,8)BTD(Q5X.Write.BDC1_Mode,0,Port_Data.Data_Transfer[1],0,8)BTD(Q5X.Write.BDC1_Hysteresis,8,Port_Data.Data_Transfer[2],0,8)BTD(Q5X.Write.BDC1_Hysteresis,0,Port_Data.Data_Transfer[3],0,8)MOV(Port,Port_Data.Data_Transfer[185])MOV(0,Port_Data.Data_Transfer[187])MOV(61,Port_Data.Data_Transfer[188])MOV(4,Port_Data.Data_Transfer[189])MOV(4,Inprocess_Index)OTL(Port_Data.Port_Write.[Port])OTL(Local_Control.11);
   95: NOP();
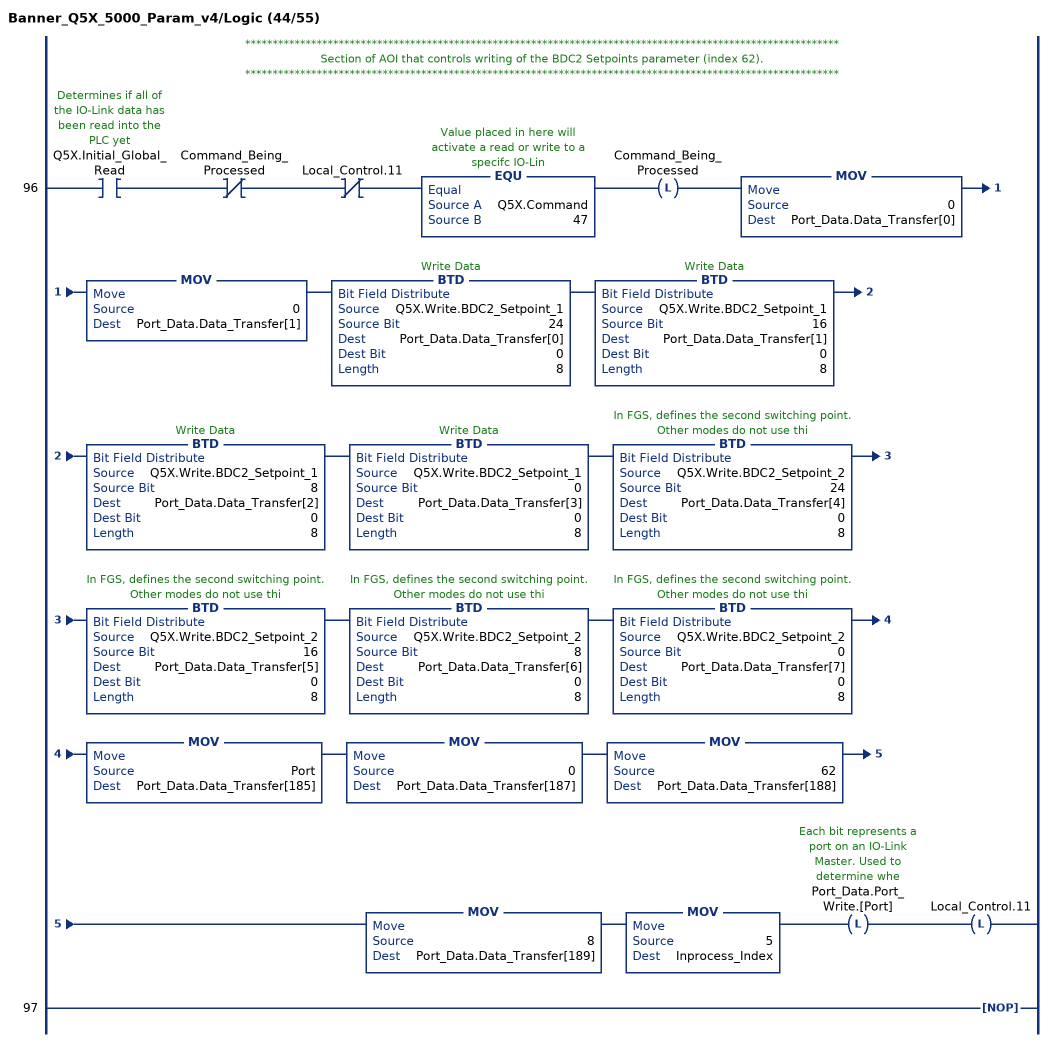
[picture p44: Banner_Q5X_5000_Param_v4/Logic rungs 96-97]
   // ************************************************************************************************************
   // Section of AOI that controls writing of the BDC2 Setpoints parameter (index 62).
   // ************************************************************************************************************
   96: XIC(Q5X.Initial_Global_Read)XIO(Command_Being_Processed)XIO(Local_Control.11)EQU(Q5X.Command,47)OTL(Command_Being_Processed)MOV(0,Port_Data.Data_Transfer[0])MOV(0,Port_Data.Data_Transfer[1])BTD(Q5X.Write.BDC2_Setpoint_1,24,Port_Data.Data_Transfer[0],0,8)BTD(Q5X.Write.BDC2_Setpoint_1,16,Port_Data.Data_Transfer[1],0,8)BTD(Q5X.Write.BDC2_Setpoint_1,8,Port_Data.Data_Transfer[2],0,8)BTD(Q5X.Write.BDC2_Setpoint_1,0,Port_Data.Data_Transfer[3],0,8)BTD(Q5X.Write.BDC2_Setpoint_2,24,Port_Data.Data_Transfer[4],0,8)BTD(Q5X.Write.BDC2_Setpoint_2,16,Port_Data.Data_Transfer[5],0,8)BTD(Q5X.Write.BDC2_Setpoint_2,8,Port_Data.Data_Transfer[6],0,8)BTD(Q5X.Write.BDC2_Setpoint_2,0,Port_Data.Data_Transfer[7],0,8)MOV(Port,Port_Data.Data_Transfer[185])MOV(0,Port_Data.Data_Transfer[187])MOV(62,Port_Data.Data_Transfer[188])MOV(8,Port_Data.Data_Transfer[189])MOV(5,Inprocess_Index)OTL(Port_Data.Port_Write.[Port])OTL(Local_Control.11);
   97: NOP();
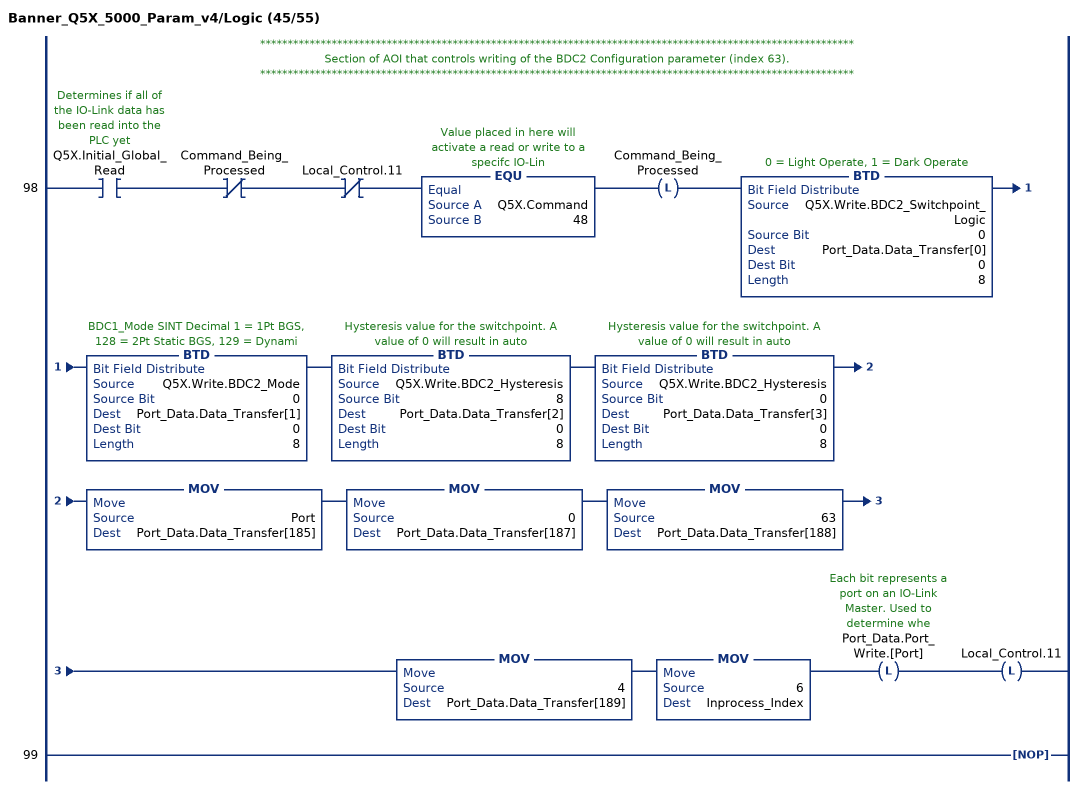
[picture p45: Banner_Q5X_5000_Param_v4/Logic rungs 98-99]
   // ************************************************************************************************************
   // Section of AOI that controls writing of the BDC2 Configuration parameter (index 63).
   // ************************************************************************************************************
   98: XIC(Q5X.Initial_Global_Read)XIO(Command_Being_Processed)XIO(Local_Control.11)EQU(Q5X.Command,48)OTL(Command_Being_Processed)BTD(Q5X.Write.BDC2_Switchpoint_Logic,0,Port_Data.Data_Transfer[0],0,8)BTD(Q5X.Write.BDC2_Mode,0,Port_Data.Data_Transfer[1],0,8)BTD(Q5X.Write.BDC2_Hysteresis,8,Port_Data.Data_Transfer[2],0,8)BTD(Q5X.Write.BDC2_Hysteresis,0,Port_Data.Data_Transfer[3],0,8)MOV(Port,Port_Data.Data_Transfer[185])MOV(0,Port_Data.Data_Transfer[187])MOV(63,Port_Data.Data_Transfer[188])MOV(4,Port_Data.Data_Transfer[189])MOV(6,Inprocess_Index)OTL(Port_Data.Port_Write.[Port])OTL(Local_Control.11);
   99: NOP();
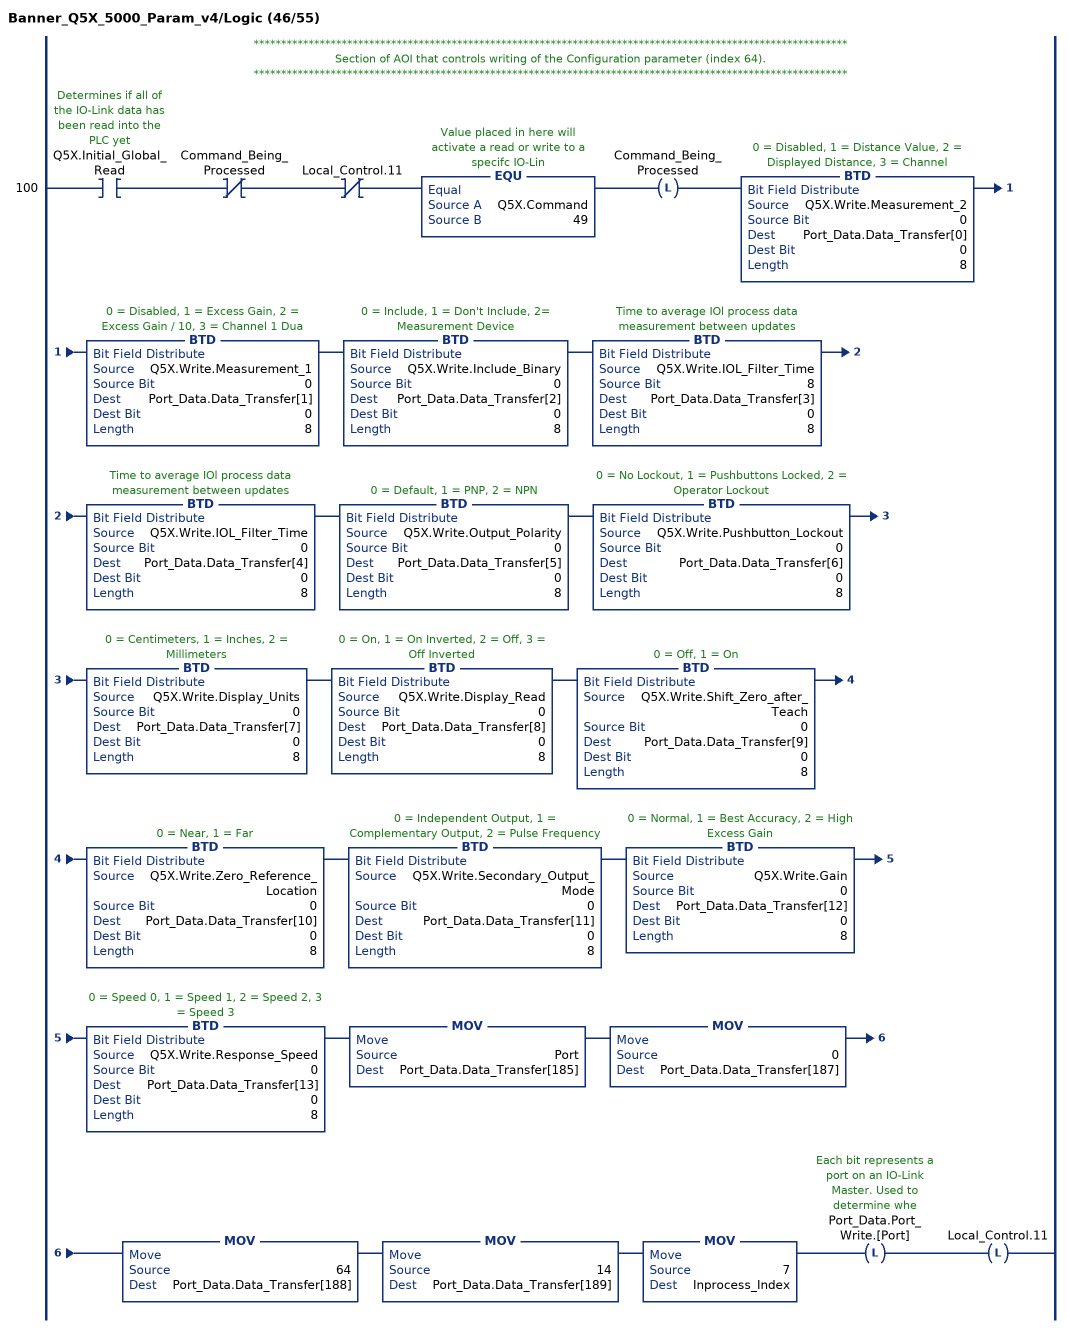
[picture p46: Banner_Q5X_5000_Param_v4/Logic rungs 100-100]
   // ************************************************************************************************************
   // Section of AOI that controls writing of the Configuration parameter (index 64).
   // ************************************************************************************************************
   100: XIC(Q5X.Initial_Global_Read)XIO(Command_Being_Processed)XIO(Local_Control.11)EQU(Q5X.Command,49)OTL(Command_Being_Processed)BTD(Q5X.Write.Measurement_2,0,Port_Data.Data_Transfer[0],0,8)BTD(Q5X.Write.Measurement_1,0,Port_Data.Data_Transfer[1],0,8)BTD(Q5X.Write.Include_Binary,0,Port_Data.Data_Transfer[2],0,8)BTD(Q5X.Write.IOL_Filter_Time,8,Port_Data.Data_Transfer[3],0,8)BTD(Q5X.Write.IOL_Filter_Time,0,Port_Data.Data_Transfer[4],0,8)BTD(Q5X.Write.Output_Polarity,0,Port_Data.Data_Transfer[5],0,8)BTD(Q5X.Write.Pushbutton_Lockout,0,Port_Data.Data_Transfer[6],0,8)BTD(Q5X.Write.Display_Units,0,Port_Data.Data_Transfer[7],0,8)BTD(Q5X.Write.Display_Read,0,Port_Data.Data_Transfer[8],0,8)BTD(Q5X.Write.Shift_Zero_after_Teach,0,Port_Data.Data_Transfer[9],0,8)BTD(Q5X.Write.Zero_Reference_Location,0,Port_Data.Data_Transfer[10],0,8)BTD(Q5X.Write.Secondary_Output_Mode,0,Port_Data.Data_Transfer[11],0,8)BTD(Q5X.Write.Gain,0,Port_Data.Data_Transfer[12],0,8)BTD(Q5X.Write.Response_Speed,0,Port_Data.Data_Transfer[13],0,8)MOV(Port,Port_Data.Data_Transfer[185])MOV(0,Port_Data.Data_Transfer[187])MOV(64,Port_Data.Data_Transfer[188])MOV(14,Port_Data.Data_Transfer[189])MOV(7,Inprocess_Index)OTL(Port_Data.Port_Write.[Port])OTL(Local_Control.11);
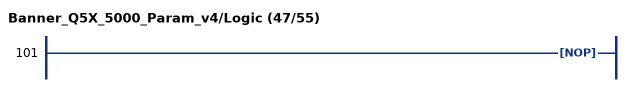
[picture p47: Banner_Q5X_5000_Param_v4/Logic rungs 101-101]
   101: NOP();
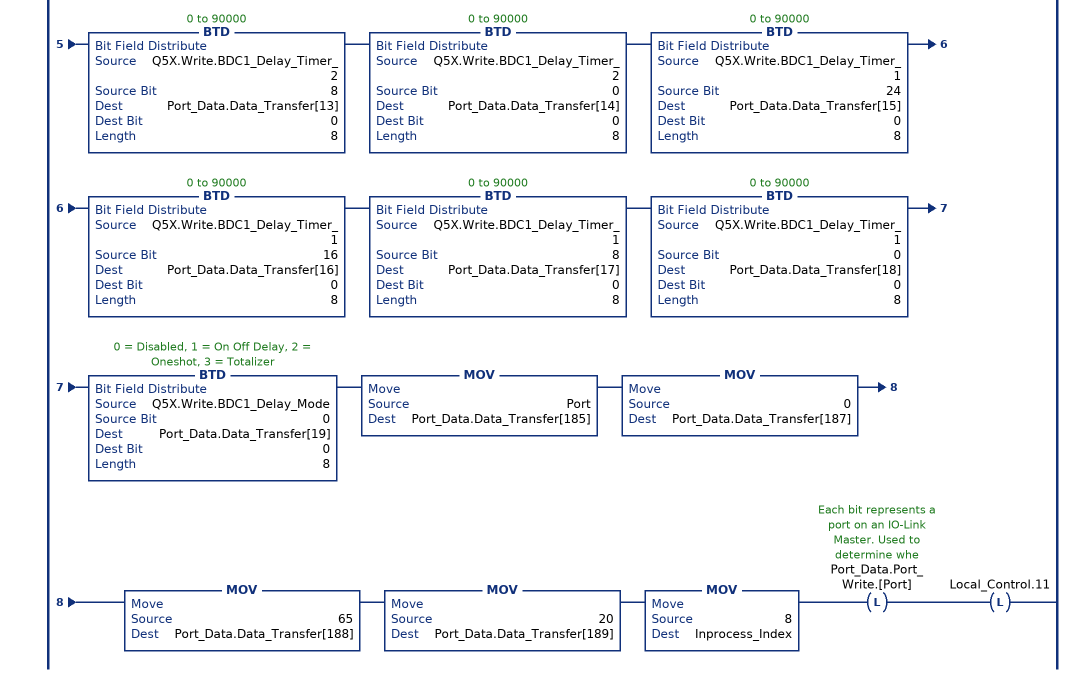
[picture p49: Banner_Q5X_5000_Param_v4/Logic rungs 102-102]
   // ************************************************************************************************************
   // Section of AOI that controls writing of the BDC1 Vendor Specific Configuration parameter (index 65).
   // ************************************************************************************************************
   102: XIC(Q5X.Initial_Global_Read)XIO(Command_Being_Processed)XIO(Local_Control.11)EQU(Q5X.Command,50)OTL(Command_Being_Processed)BTD(Q5X.Write.BDC1_Auto_Thresholding,0,Port_Data.Data_Transfer[0],0,8)BTD(Q5X.Write.BDC1_User_FGS_Window_Size,24,Port_Data.Data_Transfer[1],0,8)BTD(Q5X.Write.BDC1_User_FGS_Window_Size,16,Port_Data.Data_Transfer[2],0,8)BTD(Q5X.Write.BDC1_User_FGS_Window_Size,8,Port_Data.Data_Transfer[3],0,8)BTD(Q5X.Write.BDC1_User_FGS_Window_Size,0,Port_Data.Data_Transfer[4],0,8)BTD(Q5X.Write.BDC1_User_Teach_Offset,24,Port_Data.Data_Transfer[5],0,8)BTD(Q5X.Write.BDC1_User_Teach_Offset,16,Port_Data.Data_Transfer[6],0,8)BTD(Q5X.Write.BDC1_User_Teach_Offset,8,Port_Data.Data_Transfer[7],0,8)BTD(Q5X.Write.BDC1_User_Teach_Offset,0,Port_Data.Data_Transfer[8],0,8)BTD(Q5X.Write.BDC1_FGS_Window_Size,0,Port_Data.Data_Transfer[9],0,8)BTD(Q5X.Write.BDC1_BGS_Teach_Offset,0,Port_Data.Data_Transfer[10],0,8)BTD(Q5X.Write.BDC1_Delay_Timer_2,24,Port_Data.Data_Transfer[11],0,8)BTD(Q5X.Write.BDC1_Delay_Timer_2,16,Port_Data.Data_Transfer[12],0,8)BTD(Q5X.Write.BDC1_Delay_Timer_2,8,Port_Data.Data_Transfer[13],0,8)BTD(Q5X.Write.BDC1_Delay_Timer_2,0,Port_Data.Data_Transfer[14],0,8)BTD(Q5X.Write.BDC1_Delay_Timer_1,24,Port_Data.Data_Transfer[15],0,8)BTD(Q5X.Write.BDC1_Delay_Timer_1,16,Port_Data.Data_Transfer[16],0,8)BTD(Q5X.Write.BDC1_Delay_Timer_1,8,Port_Data.Data_Transfer[17],0,8)BTD(Q5X.Write.BDC1_Delay_Timer_1,0,Port_Data.Data_Transfer[18],0,8)BTD(Q5X.Write.BDC1_Delay_Mode,0,Port_Data.Data_Transfer[19],0,8)MOV(Port,Port_Data.Data_Transfer[185])MOV(0,Port_Data.Data_Transfer[187])MOV(65,Port_Data.Data_Transfer[188])MOV(20,Port_Data.Data_Transfer[189])MOV(8,Inprocess_Index)OTL(Port_Data.Port_Write.[Port])OTL(Local_Control.11);
